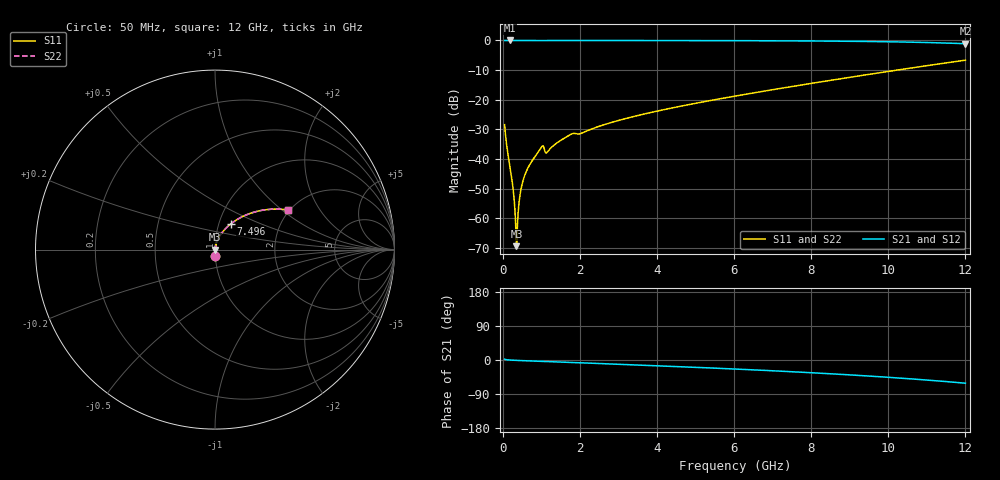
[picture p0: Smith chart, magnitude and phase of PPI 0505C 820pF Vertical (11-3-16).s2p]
# GHz S MA R 50
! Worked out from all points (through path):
!   1601 points, 50 MHz to 12 GHz, reference 50 ohm
!   highest |S21| = 0.00 dB at 191.9 MHz (marker M1); lowest = -1.1 dB at 12 GHz (marker M2)
!   group delay of S21, straight-line fit = 13.6 ps
!   lowest |S11| = -69.4 dB at 356.2 MHz (marker M3), VSWR 1.00, Z = 50 - j0.0103 ohm
!   |S11| at or under -10 dB: start of sweep to 10.23 GHz
!   |S22| runs from -69.4 to -6.7 dB; largest |S21 - S12| = 0
!   S11 on the Smith chart (normalised r, x): 50 MHz: 1.00, -0.08; 7.496 GHz: 1.14, +0.33; 12 GHz: 1.97, +1.11
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0.05  0.03801 -87.7  0.9991 2.0  0.9991 2.0  0.03801 -87.7
0.1919063  0.007241 -88.0  0.9997 -0.1  0.9997 -0.1  0.007241 -88.0
0.259125  0.003617 -85.9  0.9997 -0.5  0.9997 -0.5  0.003617 -85.9
0.318875  0.001338 -77.3  0.9997 -0.8  0.9997 -0.8  0.001338 -77.3
0.3562187  0.0003397 -17.6  0.9997 -1.0  0.9997 -1.0  0.0003397 -17.6
0.3935625  0.001044 70.0  0.9996 -1.2  0.9996 -1.2  0.001044 70.0
0.46825  0.002945 81.5  0.9996 -1.5  0.9996 -1.5  0.002945 81.5
0.5653438  0.005169 83.7  0.9996 -1.9  0.9996 -1.9  0.005169 83.7
0.70725  0.008176 84.3  0.9995 -2.5  0.9995 -2.5  0.008176 84.3
0.9835938  0.01506 79.8  0.9981 -3.7  0.9981 -3.7  0.01506 79.8
1.035875  0.01671 71.5  0.9956 -3.9  0.9956 -3.9  0.01671 71.5
1.155375  0.01308 75.4  0.9975 -4.1  0.9975 -4.1  0.01308 75.4
1.386906  0.0183 82.1  0.9988 -5.0  0.9988 -5.0  0.0183 82.1
1.737937  0.02547 79.5  0.9978 -6.5  0.9978 -6.5  0.02547 79.5
2.044156  0.02726 77.4  0.9971 -7.4  0.9971 -7.4  0.02726 77.4
2.843313  0.04183 78.1  0.998 -10.6  0.998 -10.6  0.04183 78.1
4.038312  0.06507 73.8  0.9966 -15.3  0.9966 -15.3  0.06507 73.8
6.025  0.1152 65.6  0.9917 -23.8  0.9917 -23.8  0.1152 65.6
7.496344  0.1669 58.6  0.9839 -30.9  0.9839 -30.9  0.1669 58.6
8.019156  0.1894 55.8  0.9797 -33.7  0.9797 -33.7  0.1894 55.8
10.01331  0.3014 43.8  0.9504 -45.7  0.9504 -45.7  0.3014 43.8
12  0.4646 28.3  0.8811 -61.2  0.8811 -61.2  0.4646 28.3
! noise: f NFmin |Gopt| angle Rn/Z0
0.05  0.0003042  0.8298  0.1822  0.0003764
1.372  0.003605  0.6457  3.851  0.001926
2.701  0.005311  0.5538  7.359  0.002121
4.031  0.006674  0.4926  10.58  0.002243
5.36  0.008362  0.4714  13.67  0.002647
6.682  0.01024  0.4668  16.61  0.003184
8.012  0.01242  0.4745  19.48  0.003913
9.341  0.01506  0.4933  22.32  0.004942
10.67  0.0184  0.523  25.22  0.006474
12  0.02285  0.5635  28.27  0.008907
